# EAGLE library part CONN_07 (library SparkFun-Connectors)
Multi connection point. Often used as Generic Header-pin footprint for 0.1 inch spaced/style header connections On any of the 0.1 inch spaced packages, you can populate with these: Break Away Headers - Straight (PRT-00116) Break Away Male Headers - Right Angle (PRT-00553) Female Headers (PRT-00115) Break Away Headers - Machine Pin (PRT-00117) Break Away Female Headers - Swiss Machine Pin (PRT-00743) For SCREWTERMINALS and SPRING TERMINALS visit here: Screw Terimnals on SparkFun.com (5mm/3.5mm/2.54mm spacing) This device is also useful as a general connection point to wire up your design to another part of your project. Our various solder wires solder well into these plated through hole pads. Hook-Up Wire - Assortment (Stranded, 22 AWG) (PRT-11375) Hook-Up Wire - Assortment (Solid Core, 22 AWG) (PRT-11367) View the entire wire category on our website here Special notes: Molex polarized connector foot print use with SKU : PRT-08231 with associated crimp pins and housings. 1MM SMD Version SKU: PRT-10208 NOTES ON THE VARIANTS LOCK and LOCK_LONGPADS... This footprint was designed to help hold the alignment of a through-hole component (i.e. 6-pin header) while soldering it into place. You may notice that each hole has been shifted either up or down by 0.005 of an inch from it's more standard position (which is a perfectly straight line). This slight alteration caused the pins (the squares in the middle) to touch the edges of the holes. Because they are alternating, it causes a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
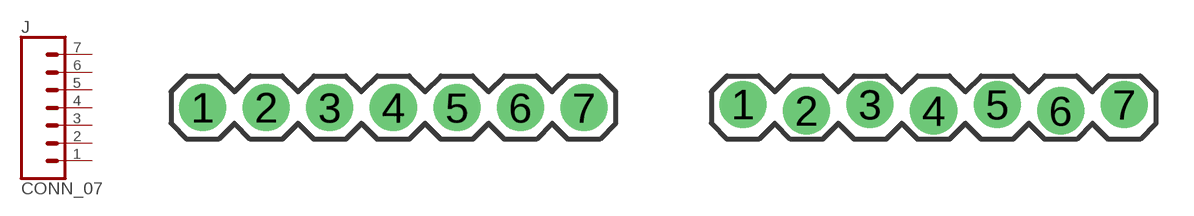
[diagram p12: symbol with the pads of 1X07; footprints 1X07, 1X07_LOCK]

Designator prefix J

## CONN_07  [1X07]
1  1  pas
2  2  pas
3  3  pas
4  4  pas
5  5  pas
6  6  pas
7  7  pas

## CONN_07LOCK  [1X07_LOCK]
Pads as for 1X07

## CONN_07LOCK_LONGPADS  [1X07_LOCK_LONGPADS]
Pads as for 1X07

## CONN_07LONGPADS  [1X07_LONGPADS]
Pads as for 1X07

## CONN_07POGOPINS_HOLES_ONLY  [1X07_HOLES_ONLY]
Pads as for 1X07

## CONN_07NO_SILK  [1X07_NO_SILK]
Pads as for 1X07

## CONN_073.5MM-7  [SCREWTERMINAL-3.5MM-7]
Pads as for 1X07

## Footprint 1X07 (pad centres in mm)
Plated Through Hole -7 Pin Specifications: Pin count:7 Pin pitch:0.1" Example device(s): CONN_07
drill 1.016 pad 1.88: 1 0,0; 2 2.54,0; 3 5.08,0; 4 7.62,0; 5 10.16,0; 6 12.7,0; 7 15.24,0

## Footprint 1X07_LOCK (pad centres in mm)
Plated Through Hole -7 Pin Locking Footprint Holes are offset 0.005" from center, locking pins in place during soldering. Specifications: Pin count:7 Pin pitch:0.1" Example device(s): CONN_07
drill 1.016 pad 1.88: 1 0,0.127; 2 2.54,-0.127; 3 5.08,0.127; 4 7.62,-0.127; 5 10.16,0.127; 6 12.7,-0.127; 7 15.24,0.127

## Footprint 1X07_LOCK_LONGPADS (pad centres in mm)
Plated Through Hole -7 Pin Locking Footprint w/ Long Pads Holes are offset 0.005" from center, locking pins in place during soldering. Specifications: Pin count:7 Pin pitch:0.1" Example device(s):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
drill 1.016 long: 1 0,0.127; 2 2.54,-0.127; 3 5.08,0.127; 4 7.62,-0.127; 5 10.16,0.127; 6 12.7,-0.127; 7 15.24,0.127

## Footprint 1X07_LONGPADS (pad centres in mm)
Plated Through Hole -7 Pin Long Pads Specifications: Pin count:7 Pin pitch:0.1" Example device(s): CONN_07
drill 1.016 pad 1.88 long: 1 0,0; 2 2.54,0; 3 5.08,0; 4 7.62,0; 5 10.16,0; 6 12.7,0; 7 15.24,0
